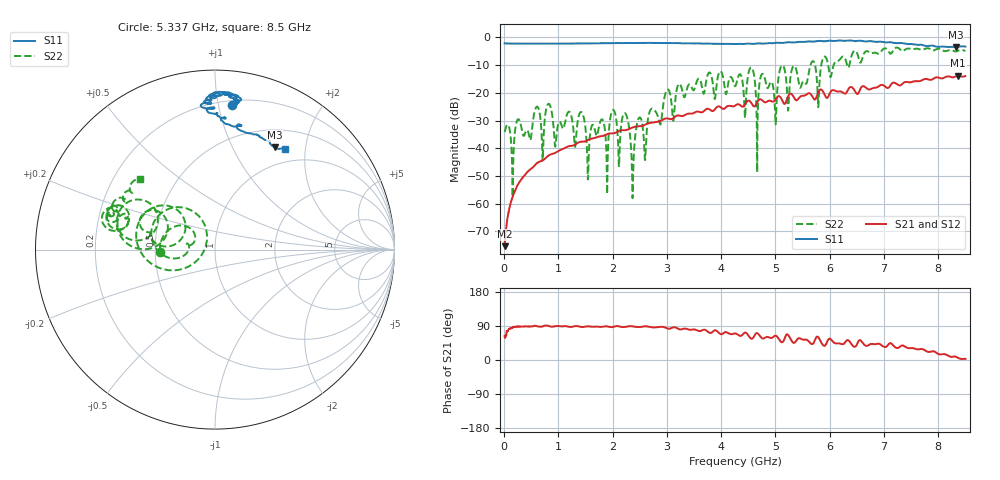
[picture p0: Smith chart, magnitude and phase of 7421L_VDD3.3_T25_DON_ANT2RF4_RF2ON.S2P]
!Agilent Technologies,E5071C,MY46417908,A.11.23
!Date: Thu Feb 25 16:17:17 2021
!Data & Calibration Information:
!Freq	S11:SOLT2(ON)	S21:SOLT2(ON)	S12:SOLT2(ON)	S22:SOLT2(ON)
!PortZ  Port1:50+j0  Port2:50+j0
!Above PortZ is port z conversion or system Z0 setting when saving the data.
!When reading, reference impedance value at option line is always used.
# Hz S dB R 50
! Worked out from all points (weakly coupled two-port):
!   1601 points, 10 MHz to 8.5 GHz, reference 50 ohm
!   highest |S21| = -13.85 dB at 8.367 GHz (marker M1); lowest = -75.3 dB at 10 MHz (marker M2)
!   lowest |S11| = -3.6 dB at 8.325 GHz (marker M3), VSWR 4.87, Z = 36.6 + j73.9 ohm
!   |S11| at or under -10 dB: nowhere
!   |S22| runs from -58.0 to -3.7 dB; largest |S21 - S12| = 0.0028
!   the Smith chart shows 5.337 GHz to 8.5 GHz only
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1e7  -2.16 179.7  -75.29 63.1  -75.23 69.8  -34.10 4.9
1.532688e8  -2.22 176.9  -57.68 86.2  -57.78 85.8  -51.82 -44.2
3.336812e8  -2.25 173.2  -50.81 88.1  -50.80 88.3  -33.87 -4.5
1.426769e9  -2.19 151.3  -37.61 87.1  -37.62 87.1  -26.97 -87.6
1.548812e9  -2.17 148.7  -36.97 88.9  -36.94 88.9  -50.72 -99.7
2.233319e9  -2.04 137.5  -33.47 87.4  -33.48 87.4  -27.43 -178.6
2.371281e9  -2.03 136.4  -32.47 88.9  -32.47 88.8  -57.34 -31.7
2.482712e9  -2.01 134.8  -32.05 86.7  -32.05 86.7  -29.18 -132.3
2.843538e9  -2.00 131.3  -30.41 86.7  -30.42 86.7  -29.15 -115.8
3.225588e9  -2.08 127.7  -28.18 81.4  -28.19 81.4  -16.75 -99.3
4.255e9  -2.39 106.7  -24.62 70.1  -24.62 70.0  -17.60 -134.6
4.557456e9  -2.31 99.4  -23.69 56.3  -23.68 56.3  -10.86 -154.4
4.997875e9  -1.99 86.9  -22.47 64.2  -22.48 64.2  -29.16 165.4
5.114612e9  -1.99 86.5  -22.27 46.8  -22.23 46.9  -10.22 -174.6
5.236656e9  -1.73 84.3  -21.15 65.5  -21.15 65.6  -26.40 -25.4
5.671769e9  -1.51 82.6  -21.04 42.1  -21.00 42.2  -8.83 168.2
5.788506e9  -1.30 81.8  -19.77 60.2  -19.78 60.4  -25.16 157.4
5.899938e9  -1.40 83.1  -20.35 37.2  -20.30 37.5  -6.94 167.0
7.088538e9  -1.72 92.0  -18.09 42.1  -18.14 41.8  -5.23 155.4
8.324894e9  -3.62 59.8  -14.03 8.7  -14.04 8.2  -5.08 145.4
8.367344e9  -3.39 56.4  -13.85 5.4  -13.87 5.1  -4.78 145.1
8.5e9  -3.34 55.0  -13.95 3.0  -14.02 2.6  -4.86 136.8
